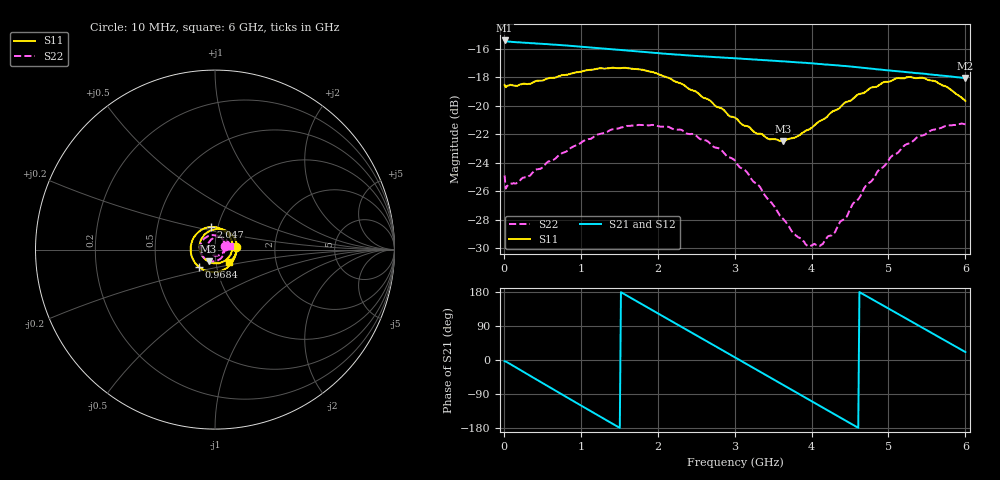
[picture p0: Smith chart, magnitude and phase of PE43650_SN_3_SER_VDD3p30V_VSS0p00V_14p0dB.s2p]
!Keysight Technologies,N5245B,MY57181451,A.13.50.07
!Date: Tuesday, May 07, 2019 08:00:13
!Correction: S11(Full 2 Port(1,2))
!S21(Full 2 Port(1,2))
!S12(Full 2 Port(1,2))
!S22(Full 2 Port(1,2))
!S2P File: Measurements: S11, S21, S12, S22:
# Hz S  dB  R 50
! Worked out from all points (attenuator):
!   401 points, 10 MHz to 6 GHz, reference 50 ohm
!   highest |S21| = -15.40 dB at 10 MHz (marker M1); lowest = -18.0 dB at 6 GHz (marker M2)
!   lowest |S11| = -22.5 dB at 3.634 GHz (marker M3), VSWR 1.16, Z = 46.2 - j6.14 ohm
!   |S11| at or under -10 dB: start of sweep to end of sweep
!   |S22| runs from -29.9 to -21.2 dB; largest |S21 - S12| = 0.0018
!   S11 on the Smith chart (normalised r, x): 10 MHz: 1.27, +0.03; 968.4 MHz: 0.82, -0.16; 2.047 GHz: 0.93, +0.24; 6 GHz: 1.16, -0.16
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1e7  -18.53 5.9  -15.40 -3.5  -15.49 -3.4  -24.89 20.2
1.44775e8  -18.58 -21.0  -15.51 -18.0  -15.56 -18.0  -25.47 -19.7
5.1915e8  -18.18 -74.5  -15.64 -62.7  -15.69 -62.7  -24.22 -73.4
7.43775e8  -17.86 -104.2  -15.73 -89.4  -15.77 -89.4  -23.38 -100.8
9.684e8  -17.63 -133.0  -15.82 -116.0  -15.86 -116.0  -22.72 -127.1
1.013325e9  -17.58 -138.8  -15.84 -121.3  -15.89 -121.3  -22.55 -132.3
1.252925e9  -17.35 -167.7  -15.94 -149.5  -16.00 -149.5  -21.96 -157.5
1.5075e9  -17.35 162.1  -16.06 -179.3  -16.12 -179.3  -21.56 176.4
1.7471e9  -17.42 134.6  -16.18 152.7  -16.23 152.7  -21.34 153.0
2.01665e9  -17.78 103.8  -16.29 121.4  -16.35 121.4  -21.44 127.4
2.0466e9  -17.86 100.2  -16.31 117.9  -16.36 117.9  -21.47 124.3
2.480875e9  -18.95 48.7  -16.48 67.6  -16.53 67.7  -22.04 82.9
3.005e9  -20.82 -19.5  -16.65 6.9  -16.71 7.0  -23.87 29.9
3.33445e9  -21.96 -69.2  -16.76 -31.3  -16.81 -31.2  -25.73 -8.1
3.63395e9  -22.47 -118.4  -16.87 -66.1  -16.91 -66.0  -27.97 -49.6
3.7837e9  -22.22 -142.9  -16.92 -83.5  -16.97 -83.4  -29.05 -73.9
4.008325e9  -21.52 -178.0  -17.01 -109.5  -17.06 -109.5  -29.80 -115.9
4.277875e9  -20.37 144.6  -17.13 -140.8  -17.18 -140.8  -29.02 -165.9
4.517475e9  -19.60 113.7  -17.24 -168.7  -17.29 -168.5  -27.10 155.5
5.01165e9  -18.28 57.8  -17.51 134.4  -17.56 134.5  -23.73 97.7
5.475875e9  -18.08 10.3  -17.74 81.0  -17.80 81.1  -22.02 54.6
6e9  -19.65 -40.6  -18.04 21.0  -18.09 21.1  -21.29 12.5
